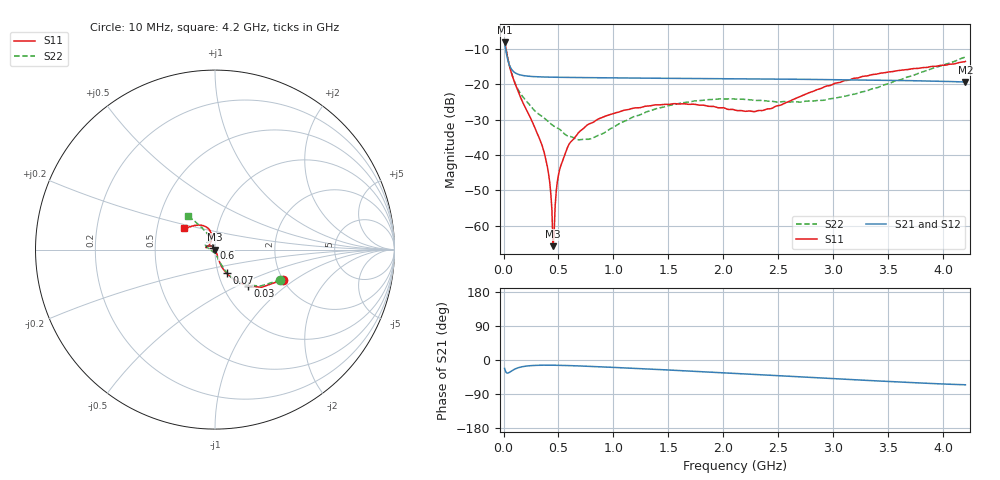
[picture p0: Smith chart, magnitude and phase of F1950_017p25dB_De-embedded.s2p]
! Integrated Device Technology
! Corporate Headquarters
! 6024 Silver Creek Valley Road
! San Jose, CA 95138  USA
! Phone:  1-408-284-8200
! Toll Free:  1-800-223-1366
! Webpage:  http://www.idt.com/
! Timing and RF Division
! 515 Groton Road, Suite 102
! Westford, MA 01886-6024
! Device:  F1950
! Description: 7-bit 0.25 dB Digital Step Attenuator
! Frequency:  150.0 -  4000.00 MHz
! Package:  4x4 mm Thin QFN Plastic Package: 24 pin
! Ports:  2 RF, 12 DC
!  Pin  1  = D0
!  Pin  2  = VDD
!  Pin  3  = Vmode
!  Pin  4  = GND
!  Pin  5  = RF1  =  Port 1
!  Pin  6  = GND
!  Pin  7  = GND
!  Pin  8  = GND
!  Pin  9  = GND
!  Pin 10  = GND
!  Pin 11  = GND
!  Pin 12  = GND
!  Pin 13  = GND
!  Pin 14  = RF2  =  Port 2
!  Pin 15  = GND
!  Pin 16  = LE
!  Pin 17  = CLK
!  Pin 18  = DATE
!  Pin 19  = D6
!  Pin 20  = D5
!  Pin 21  = D4
!  Pin 22  = D3
!  Pin 23  = D2
!  Pin 24  = D1
! State:  69
! Atten State:  17.25 dB
! Voltage:  +5.00 Volts
! Current:  Not Measured mA
! Data:  The device was measured on a the F195X evaluation board which has
!  individual transmission lines to the RF pins.  Data was collected
!  using a calibrated network analyzer.  The evaluation board was
!  de-embedded using a TRL calibration technique.
!  The reference plane is the edge of the package pin.
! Misc:  Board 2019
!  Action Tracker AT0250
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# GHz S dB R 50
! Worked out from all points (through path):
!   420 points, 10 MHz to 4.2 GHz, reference 50 ohm
!   highest |S21| = -8.21 dB at 10 MHz (marker M1); lowest = -19.4 dB at 4.2 GHz (marker M2)
!   group delay of S21, straight-line fit = 36.5 ps
!   lowest |S11| = -65.7 dB at 450 MHz (marker M3), VSWR 1.00, Z = 50 - j0.0337 ohm
!   |S11| at or under -10 dB: 22.75 MHz to end of sweep
!   |S22| runs from -35.7 to -7.9 dB; largest |S21 - S12| = 0.00018
!   S11 on the Smith chart (normalised r, x): 10 MHz: 2.00, -0.81; 30 MHz: 1.31, -0.57; 70 MHz: 1.10, -0.29; 600 MHz: 0.98, +0.02; 4.2 GHz: 0.69, +0.17
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0.01  -7.66 -23.9  -8.21 -22.2  -8.21 -22.2  -7.92 -24.8
0.03  -11.30 -47.8  -11.94 -34.3  -11.94 -34.3  -11.43 -47.6
0.07  -16.68 -63.9  -15.66 -29.4  -15.66 -29.4  -16.53 -62.8
0.16  -24.09 -69.8  -17.45 -18.4  -17.45 -18.4  -22.91 -70.1
0.36  -38.23 -61.3  -17.97 -13.7  -17.97 -13.7  -29.33 -77.0
0.41  -45.39 -60.8  -18.01 -13.7  -18.01 -13.7  -30.62 -78.0
0.42  -47.62 -61.0  -18.02 -13.7  -18.02 -13.7  -30.89 -78.8
0.44  -55.38 -57.8  -18.04 -13.7  -18.03 -13.7  -31.44 -81.2
0.45  -65.73 -40.6  -18.04 -13.8  -18.04 -13.8  -31.67 -82.6
0.47  -54.14 111.8  -18.05 -13.8  -18.05 -13.9  -32.05 -85.5
0.49  -47.40 119.0  -18.06 -14.0  -18.06 -14.0  -32.37 -87.5
0.51  -44.15 123.8  -18.07 -14.1  -18.07 -14.1  -32.74 -88.7
0.6  -36.77 129.1  -18.11 -14.8  -18.11 -14.8  -34.72 -103.3
0.71  -32.94 133.6  -18.14 -15.9  -18.14 -15.9  -35.63 -124.2
0.99  -28.34 145.1  -18.23 -19.4  -18.23 -19.4  -32.30 -172.5
1.41  -25.84 161.7  -18.34 -25.1  -18.34 -25.2  -26.75 164.9
1.74  -25.70 167.6  -18.41 -29.9  -18.40 -29.9  -24.72 156.1
2.11  -27.36 156.4  -18.49 -35.6  -18.49 -35.6  -24.24 146.6
2.43  -26.93 123.9  -18.56 -40.3  -18.56 -40.3  -24.81 136.4
2.81  -22.09 103.6  -18.66 -46.2  -18.66 -46.2  -24.80 121.1
3.51  -16.52 116.4  -18.91 -56.8  -18.91 -56.8  -19.81 116.6
4.2  -13.60 145.5  -19.39 -65.4  -19.38 -65.5  -12.33 128.7
